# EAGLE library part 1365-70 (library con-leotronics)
DUAL ROW STRAIGHT HEADER 1364 SERIES. 1.27mm x 1.27mm. Without Fixing Post. SMT Source: http://www.leotronics.co.uk/Conexcon/Data%20Sheets/sec.%20A/1364ing.pdf
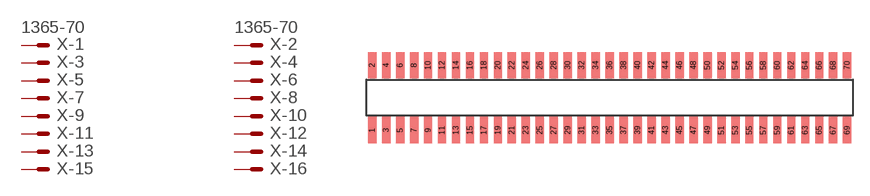
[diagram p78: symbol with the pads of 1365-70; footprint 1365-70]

Designator prefix X; gates -1=MVAL -2=MVAL -3=M -4=M -5=M -6=M -7=M -8=M -9=M -10=M -11=M -12=M -13=M -14=M -15=M -16=M -17=M -18=M -19=M -20=M -21=M -22=M -23=M -24=M -25=M -26=M -27=M -28=M -29=M -30=M -31=M -32=M -33=M -34=M -35=M -36=M -37=M -38=M -39=M -40=M -41=M -42=M -43=M -44=M -45=M -46=M -47=M -48=M -49=M -50=M -51=M -52=M -53=M -54=M -55=M -56=M -57=M -58=M -59=M -60=M -61=M -62=M -63=M -64=M -65=M -66=M -67=M -68=M -69=M -70=M

## 1365-70 (OC_FARNELL: unknown; OC_NEWARK: unknown)  [1365-70]
1  -1:S  pas
2  -2:S  pas
3  -3:S  pas
4  -4:S  pas
5  -5:S  pas
6  -6:S  pas
7  -7:S  pas
8  -8:S  pas
9  -9:S  pas
10  -10:S  pas
11  -11:S  pas
12  -12:S  pas
13  -13:S  pas
14  -14:S  pas
15  -15:S  pas
16  -16:S  pas
17  -17:S  pas
18  -18:S  pas
19  -19:S  pas
20  -20:S  pas
21  -21:S  pas
22  -22:S  pas
23  -23:S  pas
24  -24:S  pas
25  -25:S  pas
26  -26:S  pas
27  -27:S  pas
28  -28:S  pas
29  -29:S  pas
30  -30:S  pas
31  -31:S  pas
32  -32:S  pas
33  -33:S  pas
34  -34:S  pas
35  -35:S  pas
36  -36:S  pas
37  -37:S  pas
38  -38:S  pas
39  -39:S  pas
40  -40:S  pas
41  -41:S  pas
42  -42:S  pas
43  -43:S  pas
44  -44:S  pas
45  -45:S  pas
46  -46:S  pas
47  -47:S  pas
48  -48:S  pas
49  -49:S  pas
50  -50:S  pas
51  -51:S  pas
52  -52:S  pas
53  -53:S  pas
54  -54:S  pas
55  -55:S  pas
56  -56:S  pas
57  -57:S  pas
58  -58:S  pas
59  -59:S  pas
60  -60:S  pas
61  -61:S  pas
62  -62:S  pas
63  -63:S  pas
64  -64:S  pas
65  -65:S  pas
66  -66:S  pas
67  -67:S  pas
68  -68:S  pas
69  -69:S  pas
70  -70:S  pas

## Footprint 1365-70 (pad centres in mm)
DUAL ROW STRAIGHT HEADER 1364 SERIES. 1.27mm x 1.27mm. Without Fixing Post. SMT Source: http://www.leotronics.co.uk/Conexcon/Data%20Sheets/sec.%20A/1364ing.pdf
smd 0.76 x 2.4: 1 -21.59,-2.95; 2 -21.59,2.95; 3 -20.32,-2.95; 4 -20.32,2.95; 5 -19.05,-2.95; 6 -19.05,2.95; 7 -17.78,-2.95; 8 -17.78,2.95; 9 -16.51,-2.95; 10 -16.51,2.95; 11 -15.24,-2.95; 12 -15.24,2.95; 13 -13.97,-2.95; 14 -13.97,2.95; 15 -12.7,-2.95; 16 -12.7,2.95; 17 -11.43,-2.95; 18 -11.43,2.95; 19 -10.16,-2.95; 20 -10.16,2.95; 21 -8.89,-2.95; 22 -8.89,2.95; 23 -7.62,-2.95; 24 -7.62,2.95; 25 -6.35,-2.95; 26 -6.35,2.95; 27 -5.08,-2.95; 28 -5.08,2.95; 29 -3.81,-2.95; 30 -3.81,2.95; 31 -2.54,-2.95; 32 -2.54,2.95; 33 -1.27,-2.95; 34 -1.27,2.95; 35 0,-2.95; 36 0,2.95; 37 1.27,-2.95; 38 1.27,2.95; 39 2.54,-2.95; 40 2.54,2.95; 41 3.81,-2.95; 42 3.81,2.95; 43 5.08,-2.95; 44 5.08,2.95; 45 6.35,-2.95; 46 6.35,2.95; 47 7.62,-2.95; 48 7.62,2.95; 49 8.89,-2.95; 50 8.89,2.95; 51 10.16,-2.95; 52 10.16,2.95; 53 11.43,-2.95; 54 11.43,2.95; 55 12.7,-2.95; 56 12.7,2.95; 57 13.97,-2.95; 58 13.97,2.95; 59 15.24,-2.95; 60 15.24,2.95; 61 16.51,-2.95; 62 16.51,2.95; 63 17.78,-2.95; 64 17.78,2.95; 65 19.05,-2.95; 66 19.05,2.95; 67 20.32,-2.95; 68 20.32,2.95; 69 21.59,-2.95; 70 21.59,2.95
